FUNCTION_BLOCK PS_PackML_StateMachine_Auto
VAR_IN_OUT
	Machine				: Machine_REF;
END_VAR
VAR_INPUT
	Start				: BOOL;
	Hold				: BOOL;
	UnHold				: BOOL;
	Suspend				: BOOL;
	UnSuspend			: BOOL;
	Abort				: BOOL;
	Stop				: BOOL;
	Complete			: BOOL;
	Clear				: BOOL;
	Reset				: BOOL;
	StateComplete		: BOOL;
END_VAR
VAR_OUTPUT
	Status				: WORD;

	ST_Starting			: BOOL;
	ST_Completing		: BOOL;
	ST_Resetting		: BOOL;
	ST_Holding			: BOOL;
	ST_UnHolding		: BOOL;
	ST_Suspending		: BOOL;
	ST_UnSuspending		: BOOL;
	ST_Clearing			: BOOL;
	ST_Stopping			: BOOL;
	ST_Aborting			: BOOL;

	(* State Complete*)
	ST_Execute			: BOOL;
	ST_Complete			: BOOL;
	ST_Idle				: BOOL;
	ST_Held				: BOOL;
	ST_Suspended		: BOOL;
	ST_Stopped			: BOOL;
	ST_Aborted			: BOOL;

	(* additional *)
	Error				: BOOL;
	ErrorID				: DWORD;
	ePMLState			: E_PMLState := ePMLState_IDLE;
END_VAR
VAR
	ePMLStatePrev		: E_PMLState;
	bStateChange		: BOOL;
	StateCompletePrev	: BOOL;
END_VAR

(* check for state change *)
IF ePMLStatePrev <> ePMLState THEN
	ePMLStatePrev 	:= ePMLState;
	bStateChange	:= TRUE;
ELSE
	bStateChange	:= FALSE;
END_IF


(* change to new state if requested *)
CASE ePMLState OF
	ePMLState_UNDEFINED:
		(* undefined state *)
		IF bStateChange THEN
			(* transient state *)
			ST_Starting		:= FALSE;
			ST_Completing	:= FALSE;
			ST_Resetting	:= FALSE;
			ST_Holding		:= FALSE;
			ST_UnHolding	:= FALSE;
			ST_Suspending	:= FALSE;
			ST_UnSuspending	:= FALSE;
			ST_Clearing		:= FALSE;
			ST_Stopping		:= FALSE;
			ST_Aborting		:= FALSE;

			(* final state *)
			ST_Execute		:= FALSE;
			ST_Complete		:= FALSE;
			ST_Idle			:= FALSE;
			ST_Held			:= FALSE;
			ST_Suspended	:= FALSE;
			ST_Stopped		:= FALSE;
			ST_Aborted		:= FALSE;
		END_IF

		IF Abort THEN
			ePMLState 		:= ePMLState_ABORTING;
			ST_Aborting		:= TRUE;
		ELSIF Stop THEN
			ePMLState 		:= ePMLState_STOPPING;
			ST_Stopping		:= TRUE;
		END_IF


	ePMLState_IDLE:
		(* final state *)

		IF bStateChange THEN
			(* transient state *)
			ST_Starting		:= FALSE;
			ST_Completing	:= FALSE;
			ST_Resetting	:= FALSE;
			ST_Holding		:= FALSE;
			ST_UnHolding	:= FALSE;
			ST_Suspending	:= FALSE;
			ST_UnSuspending	:= FALSE;
			ST_Clearing		:= FALSE;
			ST_Stopping		:= FALSE;
			ST_Aborting		:= FALSE;

			(* final state *)
			ST_Execute		:= FALSE;
			ST_Complete		:= FALSE;
			ST_Idle			:= TRUE;
			ST_Held			:= FALSE;
			ST_Suspended	:= FALSE;
			ST_Stopped		:= FALSE;
			ST_Aborted		:= FALSE;
		END_IF

		IF Abort THEN
			ePMLState 		:= ePMLState_ABORTING;
			ST_Idle			:= FALSE;
			ST_Aborting		:= TRUE;
		ELSIF Stop THEN
			ePMLState 		:= ePMLState_STOPPING;
			ST_Idle			:= FALSE;
			ST_Stopping		:= TRUE;
		ELSIF Start THEN
			ePMLState 		:= ePMLState_STARTING;
			ST_Idle			:= FALSE;
			ST_Starting		:= TRUE;
		END_IF


	ePMLState_STARTING:
		(* transient state *)

		IF bStateChange THEN
			(* transient state *)
			ST_Starting		:= TRUE;
			ST_Completing	:= FALSE;
			ST_Resetting	:= FALSE;
			ST_Holding		:= FALSE;
			ST_UnHolding	:= FALSE;
			ST_Suspending	:= FALSE;
			ST_UnSuspending	:= FALSE;
			ST_Clearing		:= FALSE;
			ST_Stopping		:= FALSE;
			ST_Aborting		:= FALSE;

			(* final state *)
			ST_Execute		:= FALSE;
			ST_Complete		:= FALSE;
			ST_Idle			:= FALSE;
			ST_Held			:= FALSE;
			ST_Suspended	:= FALSE;
			ST_Stopped		:= FALSE;
			ST_Aborted		:= FALSE;
		END_IF

		IF Abort THEN
			ePMLState 		:= ePMLState_ABORTING;
			ST_Starting		:= FALSE;
			ST_Aborting		:= TRUE;
		ELSIF Stop THEN
			ePMLState 		:= ePMLState_STOPPING;
			ST_Starting		:= FALSE;
			ST_Stopping		:= TRUE;
		ELSIF StateComplete AND NOT StateCompletePrev THEN
			ePMLState 		:= ePMLState_EXECUTE;
			StateCompletePrev := StateComplete;
			ST_Starting		:= FALSE;
			ST_Execute		:= TRUE;
		END_IF


	ePMLState_EXECUTE:
		(* final state *)

		IF bStateChange THEN
			(* transient state *)
			ST_Starting		:= FALSE;
			ST_Completing	:= FALSE;
			ST_Resetting	:= FALSE;
			ST_Holding		:= FALSE;
			ST_UnHolding	:= FALSE;
			ST_Suspending	:= FALSE;
			ST_UnSuspending	:= FALSE;
			ST_Clearing		:= FALSE;
			ST_Stopping		:= FALSE;
			ST_Aborting		:= FALSE;

			(* final state *)
			ST_Execute		:= TRUE;
			ST_Complete		:= FALSE;
			ST_Idle			:= FALSE;
			ST_Held			:= FALSE;
			ST_Suspended	:= FALSE;
			ST_Stopped		:= FALSE;
			ST_Aborted		:= FALSE;
		END_IF

		IF Abort THEN
			ePMLState 		:= ePMLState_ABORTING;
			ST_Execute		:= FALSE;
			ST_Aborting		:= TRUE;
		ELSIF Stop THEN
			ePMLState 		:= ePMLState_STOPPING;
			ST_Execute		:= FALSE;
			ST_Stopping		:= TRUE;
		ELSIF Suspend THEN
			ePMLState 		:= ePMLState_SUSPENDING;
			ST_Execute		:= FALSE;
			ST_Suspending	:= TRUE;
		ELSIF Hold THEN
			ePMLState 		:= ePMLState_HOLDING;
			ST_Execute		:= FALSE;
			ST_Holding		:= TRUE;
		ELSIF Complete THEN
			ePMLState 		:= ePMLState_COMPLETING;
			ST_Execute		:= FALSE;
			ST_Completing	:= TRUE;
		END_IF


	ePMLState_COMPLETING:
		(* transient state *)

		IF bStateChange THEN
			(* transient state *)
			ST_Starting		:= FALSE;
			ST_Completing	:= TRUE;
			ST_Resetting	:= FALSE;
			ST_Holding		:= FALSE;
			ST_UnHolding	:= FALSE;
			ST_Suspending	:= FALSE;
			ST_UnSuspending	:= FALSE;
			ST_Clearing		:= FALSE;
			ST_Stopping		:= FALSE;
			ST_Aborting		:= FALSE;

			(* final state *)
			ST_Execute		:= FALSE;
			ST_Complete		:= FALSE;
			ST_Idle			:= FALSE;
			ST_Held			:= FALSE;
			ST_Suspended	:= FALSE;
			ST_Stopped		:= FALSE;
			ST_Aborted		:= FALSE;
		END_IF

		IF Abort THEN
			ePMLState 		:= ePMLState_ABORTING;
			ST_Completing	:= FALSE;
			ST_Aborting		:= TRUE;
		ELSIF Stop THEN
			ePMLState 		:= ePMLState_STOPPING;
			ST_Completing	:= FALSE;
			ST_Stopping		:= TRUE;
		ELSIF StateComplete AND NOT StateCompletePrev THEN
			ePMLState 		:= ePMLState_COMPLETE;
			StateCompletePrev := StateComplete;
			ST_Completing	:= FALSE;
			ST_Complete		:= TRUE;
		END_IF


	ePMLState_COMPLETE:
		(* final state *)

		IF bStateChange THEN
			(* transient state *)
			ST_Starting		:= FALSE;
			ST_Completing	:= FALSE;
			ST_Resetting	:= FALSE;
			ST_Holding		:= FALSE;
			ST_UnHolding	:= FALSE;
			ST_Suspending	:= FALSE;
			ST_UnSuspending	:= FALSE;
			ST_Clearing		:= FALSE;
			ST_Stopping		:= FALSE;
			ST_Aborting		:= FALSE;

			(* final state *)
			ST_Execute		:= FALSE;
			ST_Complete		:= TRUE;
			ST_Idle			:= FALSE;
			ST_Held			:= FALSE;
			ST_Suspended	:= FALSE;
			ST_Stopped		:= FALSE;
			ST_Aborted		:= FALSE;
		END_IF

		IF Abort THEN
			ePMLState 		:= ePMLState_ABORTING;
			ST_Complete		:= FALSE;
			ST_Aborting		:= TRUE;
		ELSIF Stop THEN
			ePMLState 		:= ePMLState_STOPPING;
			ST_Complete		:= FALSE;
			ST_Stopping		:= TRUE;
		ELSIF Reset THEN
			ePMLState 		:= ePMLState_RESETTING;
			ST_Complete		:= FALSE;
			ST_Resetting	:= TRUE;
		END_IF


	ePMLState_RESETTING:
		(* transient state *)

		IF bStateChange THEN
			(* transient state *)
			ST_Starting		:= FALSE;
			ST_Completing	:= FALSE;
			ST_Resetting	:= TRUE;
			ST_Holding		:= FALSE;
			ST_UnHolding	:= FALSE;
			ST_Suspending	:= FALSE;
			ST_UnSuspending	:= FALSE;
			ST_Clearing		:= FALSE;
			ST_Stopping		:= FALSE;
			ST_Aborting		:= FALSE;

			(* final state *)
			ST_Execute		:= FALSE;
			ST_Complete		:= FALSE;
			ST_Idle			:= FALSE;
			ST_Held			:= FALSE;
			ST_Suspended	:= FALSE;
			ST_Stopped		:= FALSE;
			ST_Aborted		:= FALSE;
		END_IF

		IF Abort THEN
			ePMLState 		:= ePMLState_ABORTING;
			ST_Resetting	:= FALSE;
			ST_Aborting		:= TRUE;
		ELSIF Stop THEN
			ePMLState 		:= ePMLState_STOPPING;
			ST_Resetting	:= FALSE;
			ST_Stopping		:= TRUE;
		ELSIF StateComplete THEN
			ePMLState 		:= ePMLState_IDLE;
			StateCompletePrev := StateComplete;
			ST_Resetting	:= FALSE;
			ST_Idle			:= TRUE;
		END_IF


	ePMLState_HOLDING:
		(* transient state *)

		IF bStateChange THEN
			(* transient state *)
			ST_Starting		:= FALSE;
			ST_Completing	:= FALSE;
			ST_Resetting	:= FALSE;
			ST_Holding		:= TRUE;
			ST_UnHolding	:= FALSE;
			ST_Suspending	:= FALSE;
			ST_UnSuspending	:= FALSE;
			ST_Clearing		:= FALSE;
			ST_Stopping		:= FALSE;
			ST_Aborting		:= FALSE;

			(* final state *)
			ST_Execute		:= FALSE;
			ST_Complete		:= FALSE;
			ST_Idle			:= FALSE;
			ST_Held			:= FALSE;
			ST_Suspended	:= FALSE;
			ST_Stopped		:= FALSE;
			ST_Aborted		:= FALSE;
		END_IF

		IF Abort THEN
			ePMLState 		:= ePMLState_ABORTING;
			ST_Holding		:= FALSE;
			ST_Aborting		:= TRUE;
		ELSIF Stop THEN
			ePMLState 		:= ePMLState_STOPPING;
			ST_Holding		:= FALSE;
			ST_Stopping		:= TRUE;
		ELSIF StateComplete AND NOT StateCompletePrev THEN
			ePMLState 		:= ePMLState_HELD;
			StateCompletePrev := StateComplete;
			ST_Holding		:= FALSE;
			ST_Held			:= TRUE;
		END_IF


	ePMLState_HELD:
		(* final state *)

		IF bStateChange THEN
			(* transient state *)
			ST_Starting		:= FALSE;
			ST_Completing	:= FALSE;
			ST_Resetting	:= FALSE;
			ST_Holding		:= FALSE;
			ST_UnHolding	:= FALSE;
			ST_Suspending	:= FALSE;
			ST_UnSuspending	:= FALSE;
			ST_Clearing		:= FALSE;
			ST_Stopping		:= FALSE;
			ST_Aborting		:= FALSE;

			(* final state *)
			ST_Execute		:= FALSE;
			ST_Complete		:= FALSE;
			ST_Idle			:= FALSE;
			ST_Held			:= TRUE;
			ST_Suspended	:= FALSE;
			ST_Stopped		:= FALSE;
			ST_Aborted		:= FALSE;
		END_IF

		IF Abort THEN
			ePMLState 		:= ePMLState_ABORTING;
			ST_Held			:= FALSE;
			ST_Aborting		:= TRUE;
		ELSIF Stop THEN
			ePMLState 		:= ePMLState_STOPPING;
			ST_Held			:= FALSE;
			ST_Stopping		:= TRUE;
		ELSIF UnHold THEN
			ePMLState 		:= ePMLState_UNHOLDING;
			ST_Held			:= FALSE;
			ST_UnHolding	:= TRUE;
		END_IF


	ePMLState_UNHOLDING:
		(* transient state *)

		IF bStateChange THEN
			(* transient state *)
			ST_Starting		:= FALSE;
			ST_Completing	:= FALSE;
			ST_Resetting	:= FALSE;
			ST_Holding		:= FALSE;
			ST_UnHolding	:= TRUE;
			ST_Suspending	:= FALSE;
			ST_UnSuspending	:= FALSE;
			ST_Clearing		:= FALSE;
			ST_Stopping		:= FALSE;
			ST_Aborting		:= FALSE;

			(* final state *)
			ST_Execute		:= FALSE;
			ST_Complete		:= FALSE;
			ST_Idle			:= FALSE;
			ST_Held			:= FALSE;
			ST_Suspended	:= FALSE;
			ST_Stopped		:= FALSE;
			ST_Aborted		:= FALSE;
		END_IF

		IF Abort THEN
			ePMLState 		:= ePMLState_ABORTING;
			ST_UnHolding	:= FALSE;
			ST_Aborting		:= TRUE;
		ELSIF Stop THEN
			ePMLState 		:= ePMLState_STOPPING;
			ST_UnHolding	:= FALSE;
			ST_Stopping		:= TRUE;
		ELSIF StateComplete AND NOT StateCompletePrev THEN
			ePMLState 		:= ePMLState_EXECUTE;
			StateCompletePrev := StateComplete;
			ST_UnHolding	:= FALSE;
			ST_Execute		:= TRUE;
		END_IF


	ePMLState_SUSPENDING:
		(* transient state *)

		IF bStateChange THEN
			(* transient state *)
			ST_Starting		:= FALSE;
			ST_Completing	:= FALSE;
			ST_Resetting	:= FALSE;
			ST_Holding		:= FALSE;
			ST_UnHolding	:= FALSE;
			ST_Suspending	:= TRUE;
			ST_UnSuspending	:= FALSE;
			ST_Clearing		:= FALSE;
			ST_Stopping		:= FALSE;
			ST_Aborting		:= FALSE;

			(* final state *)
			ST_Execute		:= FALSE;
			ST_Complete		:= FALSE;
			ST_Idle			:= FALSE;
			ST_Held			:= FALSE;
			ST_Suspended	:= FALSE;
			ST_Stopped		:= FALSE;
			ST_Aborted		:= FALSE;
		END_IF

		IF Abort THEN
			ePMLState 		:= ePMLState_ABORTING;
			ST_Suspending	:= FALSE;
			ST_Aborting		:= TRUE;
		ELSIF Stop THEN
			ePMLState 		:= ePMLState_STOPPING;
			ST_Suspending	:= FALSE;
			ST_Stopping		:= TRUE;
		ELSIF StateComplete AND NOT StateCompletePrev THEN
			ePMLState 		:= ePMLState_SUSPENDED;
			StateCompletePrev := StateComplete;
			ST_Suspending	:= FALSE;
			ST_Suspended	:= TRUE;
		END_IF


	ePMLState_SUSPENDED:
		(* final state *)

		IF bStateChange THEN
			(* transient state *)
			ST_Starting		:= FALSE;
			ST_Completing	:= FALSE;
			ST_Resetting	:= FALSE;
			ST_Holding		:= FALSE;
			ST_UnHolding	:= FALSE;
			ST_Suspending	:= FALSE;
			ST_UnSuspending	:= FALSE;
			ST_Clearing		:= FALSE;
			ST_Stopping		:= FALSE;
			ST_Aborting		:= FALSE;

			(* final state *)
			ST_Execute		:= FALSE;
			ST_Complete		:= FALSE;
			ST_Idle			:= FALSE;
			ST_Held			:= FALSE;
			ST_Suspended	:= TRUE;
			ST_Stopped		:= FALSE;
			ST_Aborted		:= FALSE;
		END_IF

		IF Abort THEN
			ePMLState 		:= ePMLState_ABORTING;
			ST_Suspended	:= FALSE;
			ST_Aborting		:= TRUE;
		ELSIF Stop THEN
			ePMLState 		:= ePMLState_STOPPING;
			ST_Suspended	:= FALSE;
			ST_Stopping		:= TRUE;
		ELSIF UnSuspend THEN
			ePMLState 		:= ePMLState_UNSUSPENDING;
			ST_Suspended	:= FALSE;
			ST_UnSuspending	:= TRUE;
		END_IF


	ePMLState_UNSUSPENDING:
		(* transient state *)

		IF bStateChange THEN
			(* transient state *)
			ST_Starting		:= FALSE;
			ST_Completing	:= FALSE;
			ST_Resetting	:= FALSE;
			ST_Holding		:= FALSE;
			ST_UnHolding	:= FALSE;
			ST_Suspending	:= FALSE;
			ST_UnSuspending	:= TRUE;
			ST_Clearing		:= FALSE;
			ST_Stopping		:= FALSE;
			ST_Aborting		:= FALSE;

			(* final state *)
			ST_Execute		:= FALSE;
			ST_Complete		:= FALSE;
			ST_Idle			:= FALSE;
			ST_Held			:= FALSE;
			ST_Suspended	:= FALSE;
			ST_Stopped		:= FALSE;
			ST_Aborted		:= FALSE;
		END_IF

		IF Abort THEN
			ePMLState 		:= ePMLState_ABORTING;
			ST_UnSuspending	:= FALSE;
			ST_Aborting		:= TRUE;
		ELSIF Stop THEN
			ePMLState 		:= ePMLState_STOPPING;
			ST_UnSuspending	:= FALSE;
			ST_Stopping		:= TRUE;
		ELSIF StateComplete AND NOT StateCompletePrev THEN
			ePMLState 		:= ePMLState_EXECUTE;
			StateCompletePrev := StateComplete;
			ST_UnSuspending	:= FALSE;
			ST_Execute		:= TRUE;
		END_IF


	ePMLState_STOPPING:
		(* transient state *)

		IF bStateChange THEN
			(* transient state *)
			ST_Starting		:= FALSE;
			ST_Completing	:= FALSE;
			ST_Resetting	:= FALSE;
			ST_Holding		:= FALSE;
			ST_UnHolding	:= FALSE;
			ST_Suspending	:= FALSE;
			ST_UnSuspending	:= FALSE;
			ST_Clearing		:= FALSE;
			ST_Stopping		:= TRUE;
			ST_Aborting		:= FALSE;

			(* final state *)
			ST_Execute		:= FALSE;
			ST_Complete		:= FALSE;
			ST_Idle			:= FALSE;
			ST_Held			:= FALSE;
			ST_Suspended	:= FALSE;
			ST_Stopped		:= FALSE;
			ST_Aborted		:= FALSE;
		END_IF

		IF Abort THEN
			ePMLState 		:= ePMLState_ABORTING;
			ST_Stopping		:= FALSE;
			ST_Aborting		:= TRUE;
		ELSIF StateComplete AND NOT StateCompletePrev THEN
			ePMLState 		:= ePMLState_STOPPED;
			StateCompletePrev := StateComplete;
			ST_Stopping		:= FALSE;
			ST_Stopped		:= TRUE;
		END_IF


	ePMLState_STOPPED:
		(* final state *)

		IF bStateChange THEN
			(* transient state *)
			ST_Starting		:= FALSE;
			ST_Completing	:= FALSE;
			ST_Resetting	:= FALSE;
			ST_Holding		:= FALSE;
			ST_UnHolding	:= FALSE;
			ST_Suspending	:= FALSE;
			ST_UnSuspending	:= FALSE;
			ST_Clearing		:= FALSE;
			ST_Stopping		:= FALSE;
			ST_Aborting		:= FALSE;

			(* final state *)
			ST_Execute		:= FALSE;
			ST_Complete		:= FALSE;
			ST_Idle			:= FALSE;
			ST_Held			:= FALSE;
			ST_Suspended	:= FALSE;
			ST_Stopped		:= TRUE;
			ST_Aborted		:= FALSE;
		END_IF

		IF Abort THEN
			ePMLState 		:= ePMLState_ABORTING;
			ST_Stopped		:= FALSE;
			ST_Aborting		:= TRUE;
		ELSIF Reset THEN
			ePMLState 		:= ePMLState_RESETTING;
			ST_Stopped		:= FALSE;
			ST_Resetting	:= TRUE;
		END_IF


ePMLState_ABORTING:
		(* transient state *)

		IF bStateChange THEN
			(* transient state *)
			ST_Starting		:= FALSE;
			ST_Completing	:= FALSE;
			ST_Resetting	:= FALSE;
			ST_Holding		:= FALSE;
			ST_UnHolding	:= FALSE;
			ST_Suspending	:= FALSE;
			ST_UnSuspending	:= FALSE;
			ST_Clearing		:= FALSE;
			ST_Stopping		:= FALSE;
			ST_Aborting		:= TRUE;

			(* final state *)
			ST_Execute		:= FALSE;
			ST_Complete		:= FALSE;
			ST_Idle			:= FALSE;
			ST_Held			:= FALSE;
			ST_Suspended	:= FALSE;
			ST_Stopped		:= FALSE;
			ST_Aborted		:= FALSE;
		END_IF

		IF StateComplete AND NOT StateCompletePrev THEN
			ePMLState 		:= ePMLState_ABORTED;
			StateCompletePrev := StateComplete;
			ST_Aborting		:= FALSE;
			ST_Aborted		:= TRUE;
		END_IF


	ePMLState_ABORTED:
		(* final state *)

		IF bStateChange THEN
			(* transient state *)
			ST_Starting		:= FALSE;
			ST_Completing	:= FALSE;
			ST_Resetting	:= FALSE;
			ST_Holding		:= FALSE;
			ST_UnHolding	:= FALSE;
			ST_Suspending	:= FALSE;
			ST_UnSuspending	:= FALSE;
			ST_Clearing		:= FALSE;
			ST_Stopping		:= FALSE;
			ST_Aborting		:= FALSE;

			(* final state *)
			ST_Execute		:= FALSE;
			ST_Complete		:= FALSE;
			ST_Idle			:= FALSE;
			ST_Held			:= FALSE;
			ST_Suspended	:= FALSE;
			ST_Stopped		:= FALSE;
			ST_Aborted		:= TRUE;
		END_IF

		IF Clear THEN
			ePMLState 		:= ePMLState_CLEARING;
			ST_Aborted		:= FALSE;
			ST_Clearing		:= TRUE;
		END_IF


	ePMLState_CLEARING:
		(* transient state *)

		IF bStateChange THEN
			(* transient state *)
			ST_Starting		:= FALSE;
			ST_Completing	:= FALSE;
			ST_Resetting	:= FALSE;
			ST_Holding		:= FALSE;
			ST_UnHolding	:= FALSE;
			ST_Suspending	:= FALSE;
			ST_UnSuspending	:= FALSE;
			ST_Clearing		:= TRUE;
			ST_Stopping		:= FALSE;
			ST_Aborting		:= FALSE;

			(* final state *)
			ST_Execute		:= FALSE;
			ST_Complete		:= FALSE;
			ST_Idle			:= FALSE;
			ST_Held			:= FALSE;
			ST_Suspended	:= FALSE;
			ST_Stopped		:= FALSE;
			ST_Aborted		:= FALSE;
		END_IF

		IF Abort THEN
			ePMLState 		:= ePMLState_ABORTING;
			ST_Stopped		:= FALSE;
			ST_Aborting		:= TRUE;
		ELSIF StateComplete AND NOT StateCompletePrev THEN
			ePMLState 		:= ePMLState_STOPPED;
			StateCompletePrev := StateComplete;
			ST_Clearing		:= FALSE;
			ST_Stopped		:= TRUE;
		END_IF

END_CASE

(* auto clear with StateComplete = FALSE *)
StateCompletePrev := StateCompletePrev AND StateComplete;

END_FUNCTION_BLOCK
